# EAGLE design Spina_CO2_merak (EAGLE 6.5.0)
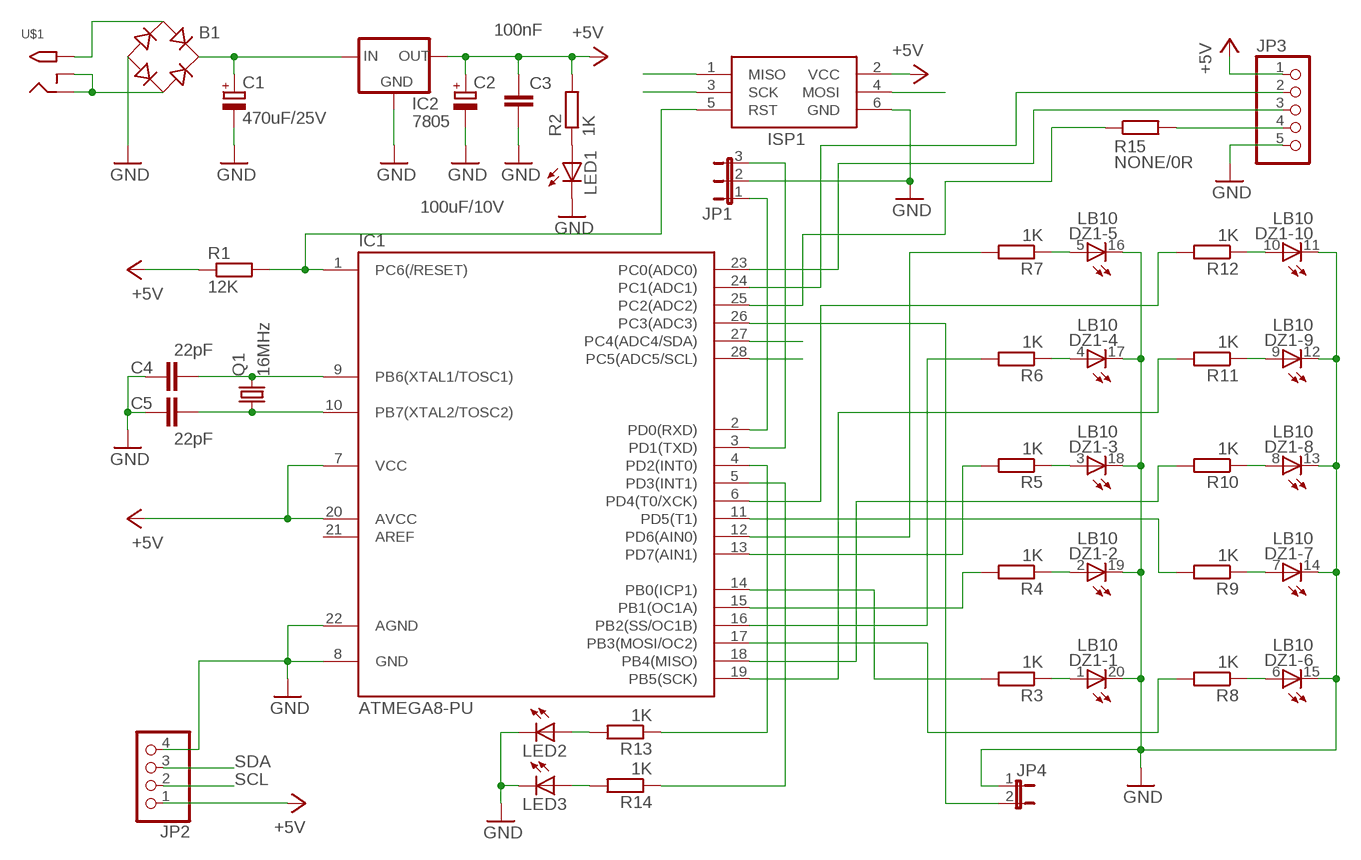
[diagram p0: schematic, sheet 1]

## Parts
B1  B-DIL  [B-DIL]
C1  470uF/25V  CPOL-EUE3.5-8  [E3,5-8]
C2  100uF/10V  CPOL-EUE2.5-6  [E2,5-6]
C3  100nF  C-EUC025_050-024X070  [C025_050-024X070]
C4  22pF  C-EUC025_050-024X070  [C025_050-024X070]
C5  22pF  C-EUC025_050-024X070  [C025_050-024X070]
DZ1  LB10  [LB10]
IC1  ATMEGA8-PU  [DIL28-3]
IC2  7805  78XXL  [78XXL]
ISP1  AVRISP-6  [AVRISP]
JP1  JP2E  [JP2]
JP2  PINHD-1X4  [1X04]
JP3  PINHD-1X5  [1X05]
JP4  JP1E  [JP1]
LED1  LED3MM  [LED3MM]
LED2  LED3MM  [LED3MM]
LED3  LED3MM  [LED3MM]
Q1  16MHz  CRYSTALHC49S  [HC49/S]
R1  12K  R-EU_0207/10  [0207/10]
R2  1K  R-EU_0207/10  [0207/10]
R3  1K  R-EU_0207/10  [0207/10]
R4  1K  R-EU_0207/10  [0207/10]
R5  1K  R-EU_0207/10  [0207/10]
R6  1K  R-EU_0207/10  [0207/10]
R7  1K  R-EU_0207/10  [0207/10]
R8  1K  R-EU_0207/10  [0207/10]
R9  1K  R-EU_0207/10  [0207/10]
R10  1K  R-EU_0207/10  [0207/10]
R11  1K  R-EU_0207/10  [0207/10]
R12  1K  R-EU_0207/10  [0207/10]
R13  1K  R-EU_0207/10  [0207/10]
R14  1K  R-EU_0207/10  [0207/10]
R15  NONE/0R  R-EU_R1206  [R1206]
U$1  2.1MMJACKTHM  [PJ-102A]

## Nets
+5V: C2.+ C3.1 IC1.7(VCC) IC1.20(AVCC) IC2.OUT ISP1.2(VCC) JP2.1 JP3.1 R1.1 R2.2
GND: B1.- C1.- C2.- C3.2 C4.1 C5.1 DZ1.11(-10:C) DZ1.12(-9:C) DZ1.13(-8:C) DZ1.14(-7:C) DZ1.15(-6:C) DZ1.16(-5:C) DZ1.17(-4:C) DZ1.18(-3:C) DZ1.19(-2:C) DZ1.20(-1:C) IC1.8(GND) IC1.22(AGND) IC2.GND ISP1.6(GND) JP1.2 JP2.4 JP3.5 JP4.1 LED1.K(C) LED2.K(C) LED3.K(C)
MISO: IC1.18(PB4(MISO)) ISP1.1(MISO) R10.2
MOSI: IC1.17(PB3(MOSI/OC2)) ISP1.4(MOSI) R8.2
N$1: B1.AC1 U$1.TIP
N$2: B1.AC2 U$1.RING U$1.RING_SW
N$3: B1.+ C1.+ IC2.IN
N$4: C4.2 IC1.9(PB6(XTAL1/TOSC1)) Q1.2
N$5: C5.2 IC1.10(PB7(XTAL2/TOSC2)) Q1.1
N$6: DZ1.5(-5:A) R7.1
N$7: IC1.1(PC6(/RESET)) ISP1.5(RST) R1.2
N$8: DZ1.10(-10:A) R12.1
N$9: LED1.A R2.1
N$10: IC1.2(PD0(RXD)) JP1.1
N$11: IC1.3(PD1(TXD)) JP1.3
N$12: DZ1.9(-9:A) R11.1
N$13: DZ1.8(-8:A) R10.1
N$14: DZ1.7(-7:A) R9.1
N$15: DZ1.2(-2:A) R4.1
N$16: DZ1.3(-3:A) R5.1
N$17: DZ1.4(-4:A) R6.1
N$18: DZ1.6(-6:A) R8.1
N$19: DZ1.1(-1:A) R3.1
N$20: IC1.24(PC1(ADC1)) JP3.2
N$21: IC1.23(PC0(ADC0)) JP3.3
N$22: IC1.25(PC2(ADC2)) R15.1
N$23: IC1.16(PB2(SS/OC1B)) R6.2
N$24: IC1.14(PB0(ICP1)) R3.2
N$25: IC1.15(PB1(OC1A)) R4.2
N$26: IC1.13(PD7(AIN1)) R5.2
N$27: IC1.11(PD5(T1)) R9.2
N$28: IC1.12(PD6(AIN0)) R7.2
N$29: IC1.6(PD4(T0/XCK)) R12.2
N$30: JP3.4 R15.2
N$31: IC1.26(PC3(ADC3)) JP4.2
N$33: LED2.A R13.2
N$34: LED3.A R14.2
N$35: IC1.4(PD2(INT0)) R13.1
N$36: IC1.5(PD3(INT1)) R14.1
SCK: IC1.19(PB5(SCK)) ISP1.3(SCK) R11.2
SCL: IC1.28(PC5(ADC5/SCL)) JP2.2
SDA: IC1.27(PC4(ADC4/SDA)) JP2.3
Unconnected: IC1.21(AREF)

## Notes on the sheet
- SDA
- SCL

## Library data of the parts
B1 = rectifier:B-DIL: RECTIFIER
C1 C2 = rcl:CPOL-EU: POLARIZED CAPACITOR, European symbol
C3-C5 = rcl:C-EU: CAPACITOR, European symbol
DZ1 = led:LB10: LED BLOCK 10-LED bar graph, DIL, Siemens
IC1 = atmega8:ATMEGA8-PU
IC2 = v-reg:78XXL: VOLTAGE REGULATOR
ISP1 = adafruit:AVRISP: AVR ISP HEADER Standard 6 pin header for AVR programming
JP1 = jumper:JP2E: JUMPER
JP2 = pinhead:PINHD-1X4: PIN HEADER
JP3 = pinhead:PINHD-1X5: PIN HEADER
JP4 = jumper:JP1E: JUMPER
LED1-LED3 = led:LED: LED
Q1 = crystal:CRYSTAL: CRYSTAL; OC_FARNELL: 1667008; OC_NEWARK: unknown
R1-R15 = rcl:R-EU_: RESISTOR, European symbol
U$1 = adafruit:2.1MMJACK: 2.1mm x 5.5mm THM DC jack with internal switch. Digikey part #PJ-102A, 4UCON part #05537 2.1mm x 5.5mm SMT DC jack with internal switch. Digikey part #PJ-002A-SMT, 4UCON part #03267 By microbuilder.eu & adafruit.com

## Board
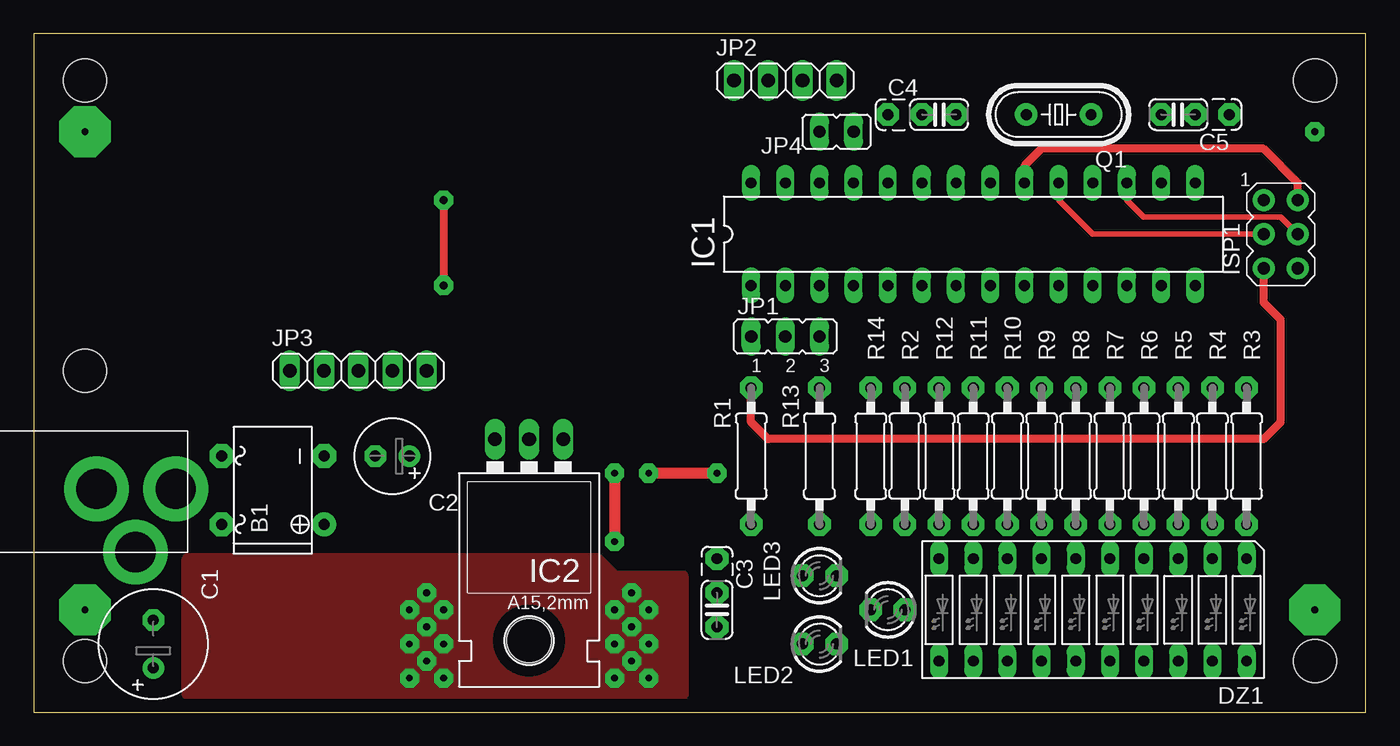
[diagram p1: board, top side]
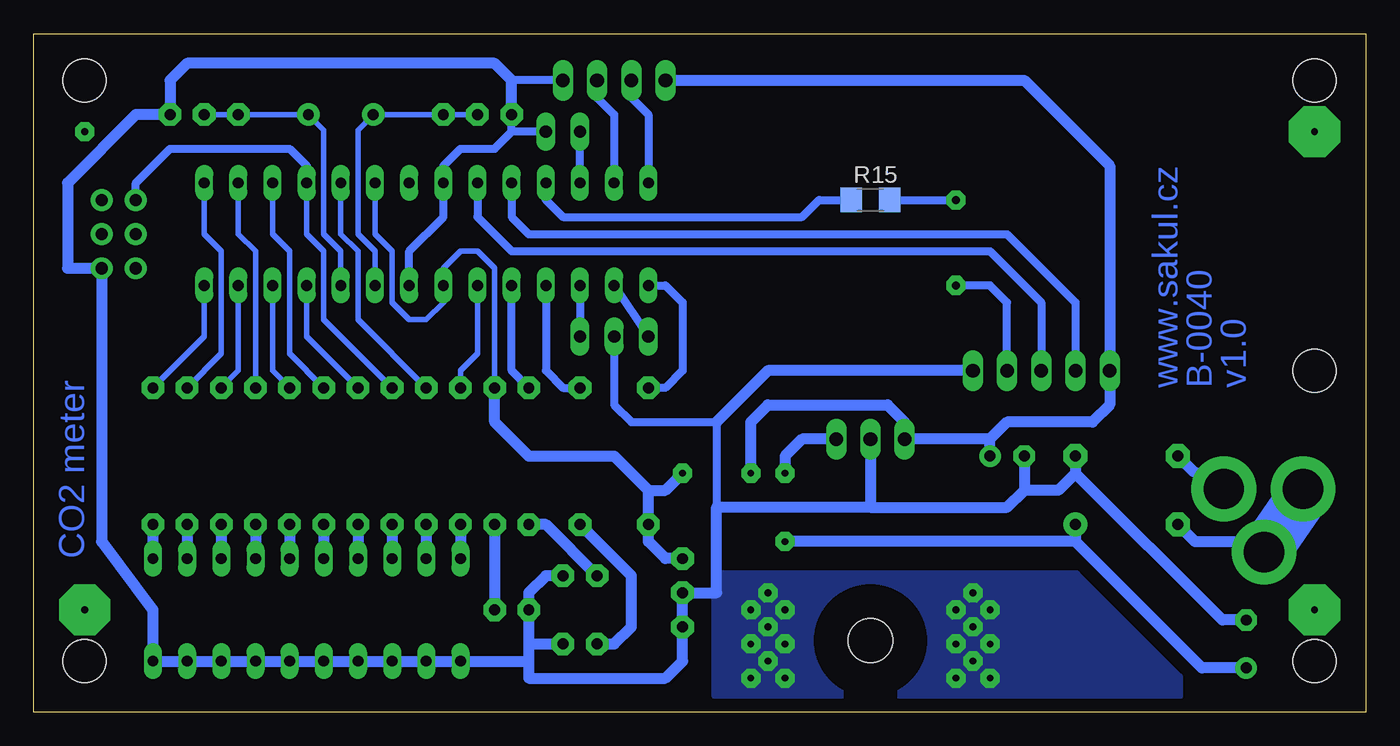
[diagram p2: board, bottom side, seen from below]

Size 99.04 x 50.47 mm. Coordinates in mm from the lower left corner, seen from the top.
Outline: 0,0 99.04,0 99.04,50.47 0,50.47 0,0
Copper layers (1*16): Top 0.035mm / dielectric 1.5mm / Bottom 0.035mm
Design rules "default": minimum track width 10mil, minimum drill 24mil, track to track 8mil, track to pad 8mil, pad to pad 8mil, via to via 8mil, smd to smd 8mil, copper to edge 40mil, drill to drill 8mil, minimum pad ring 10mil, minimum via ring 8mil, stop-mask expansion 4mil, vias tented up to drill 0mil, thermal gap 10mil
Holes 3.2 mm at 3.81,3.81 95.25,3.81 95.25,46.99 3.81,46.99 3.81,25.4

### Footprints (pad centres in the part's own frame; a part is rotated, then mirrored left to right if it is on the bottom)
B-DIL = drill 0.813 pad 1.778: + -2.54,-3.81 | drill 0.813 pad 1.778 octagon: - 2.54,-3.81; AC1 2.54,3.81; AC2 -2.54,3.81
E3,5-8 = drill 0.813 pad 1.6: + -1.778,0 | drill 0.813 pad 1.6 octagon: - 1.778,0
E2,5-6 = drill 0.813 pad 1.6: + -1.27,0 | drill 0.813 pad 1.6 octagon: - 1.27,0
C025_050-024X070 = drill 0.813 pad 1.676 octagon: 1 -3.81,0; 2 -1.27,0; 3 1.27,0
LB10 = drill 0.813 long: 1 -11.43,-3.81; 2 -8.89,-3.81; 3 -6.35,-3.81; 4 -3.81,-3.81; 5 -1.27,-3.81; 6 1.27,-3.81; 7 3.81,-3.81; 8 6.35,-3.81; 9 8.89,-3.81; 10 11.43,-3.81; 11 11.43,3.81; 12 8.89,3.81; 13 6.35,3.81; 14 3.81,3.81; 15 1.27,3.81; 16 -1.27,3.81; 17 -3.81,3.81; 18 -6.35,3.81; 19 -8.89,3.81; 20 -11.43,3.81
DIL28-3 = drill 0.813 long: 1 -16.51,-3.81; 2 -13.97,-3.81; 3 -11.43,-3.81; 4 -8.89,-3.81; 5 -6.35,-3.81; 6 -3.81,-3.81; 7 -1.27,-3.81; 8 1.27,-3.81; 9 3.81,-3.81; 10 6.35,-3.81; 11 8.89,-3.81; 12 11.43,-3.81; 13 13.97,-3.81; 14 16.51,-3.81; 15 16.51,3.81; 16 13.97,3.81; 17 11.43,3.81; 18 8.89,3.81; 19 6.35,3.81; 20 3.81,3.81; 21 1.27,3.81; 22 -1.27,3.81; 23 -3.81,3.81; 24 -6.35,3.81; 25 -8.89,3.81; 26 -11.43,3.81; 27 -13.97,3.81; 28 -16.51,3.81
78XXL = drill 1.016 long: GND 0,-3.81; IN -2.54,-3.81; OUT 2.54,-3.81 | hole 3.302: 0,11.176
AVRISP = drill 0.9 pad 1.626: 1 -1.27,2.54; 2 1.27,2.54; 3 -1.27,0; 4 1.27,0; 5 -1.27,-2.54; 6 1.27,-2.54
JP2 = drill 0.914 long: 1 -2.54,0; 2 0,0; 3 2.54,0
1X04 = drill 1.016 long: 1 -3.81,0; 2 -1.27,0; 3 1.27,0; 4 3.81,0
1X05 = drill 1.016 long: 1 -5.08,0; 2 -2.54,0; 3 0,0; 4 2.54,0; 5 5.08,0
JP1 = drill 0.914 long: 1 0,-1.27; 2 0,1.27
LED3MM = drill 0.813 pad 1.676 octagon: A -1.27,0; K 1.27,0
HC49/S = drill 0.813 pad 1.676: 1 -2.413,0; 2 2.413,0
0207/10 = drill 0.813 pad 1.676 octagon: 1 -5.08,0; 2 5.08,0
R1206 = smd 1.6 x 1.803: 1 -1.422,0; 2 1.422,0
PJ-102A = drill 3 pad 4.8: RING 0.1,-3.39; RING_SW -4.6,-6.29; TIP 0.1,-9.29

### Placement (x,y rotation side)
B1  17.78,16.51 90 top
C1  8.89,5.08 90 top
C2  26.67,19.05 180 top
C3  50.8,7.62 270 top
C4  67.31,44.45 0 top
C5  85.09,44.45 180 top
DZ1  78.74,7.62 180 top
IC1  69.85,35.56 0 top
IC2  36.83,16.51 180 top
ISP1  92.71,35.56 0 top
JP1  55.88,27.94 0 top
JP2  55.88,46.99 0 top
JP3  24.13,25.4 0 top
JP4  59.69,43.18 90 top
LED1  63.5,7.62 180 top
LED2  58.42,5.08 0 top
LED3  58.42,10.16 0 top
Q1  76.2,44.45 180 top
R1  53.34,19.05 90 top
R2  64.77,19.05 90 top
R3  90.17,19.05 90 top
R4  87.63,19.05 90 top
R5  85.09,19.05 90 top
R6  82.55,19.05 90 top
R7  80.01,19.05 90 top
R8  77.47,19.05 90 top
R9  74.93,19.05 90 top
R10  72.39,19.05 90 top
R11  69.85,19.05 90 top
R12  67.31,19.05 90 top
R13  58.42,19.05 270 top
R14  62.23,19.05 270 top
R15  36.83,38.1 0 bottom
U$1  1.27,16.51 90 top

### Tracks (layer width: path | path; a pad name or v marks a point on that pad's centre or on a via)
+5V  (via drill 0.5 pad 1.42)
  Top 0.61: ISP1.2 93.98,39.37 91.44,41.91 74.93,41.91 73.66,40.64 IC1.20
  Top 0.813: v50.8,17.78 v45.72,17.78
  Bottom 0.406: IC1.20 73.66,35.56 72.39,34.29 72.39,30.48 71.12,29.21 69.85,29.21 68.58,30.48 IC1.7 68.58,33.02 67.31,34.29 66.04,34.29 64.77,33.02 64.77,21.59
  Bottom 0.813: R2.2 64.77,21.59 62.23,19.05 55.88,19.05 53.34,16.51 | JP2.1 25.4,46.99 19.05,40.64 JP3.1 19.05,22.86 20.32,21.59 26.67,21.59 27.94,20.32 | C2.+ 27.94,20.32 | 27.94,20.32 IC2.OUT 34.29,21.59 35.56,22.86 44.45,22.86 45.72,21.59 v45.72,17.78 | C3.1 52.07,11.43 53.34,12.7 R1.1 53.34,16.51 | 53.34,16.51 52.07,16.51 v50.8,17.78
GND  (via drill 0.5 pad 1.42)
  Bottom 0.61: 63.5,43.18 64.77,41.91 67.31,41.91 68.58,40.64 IC1.22 68.58,36.83 71.12,34.29 IC1.8 | 63.5,43.18 C4.1 | JP4.1 63.5,43.18 | JP2.4 63.5,46.99 | JP1.2 55.88,22.86 54.61,21.59 48.26,21.59 48.26,15.24
  Bottom 0.813: 62.23,3.81 DZ1.11 DZ1.12 DZ1.13 DZ1.14 DZ1.15 DZ1.16 DZ1.17 DZ1.18 DZ1.19 DZ1.20 90.17,7.62 93.98,12.7 ISP1.6 96.52,33.02 96.52,39.37 91.44,44.45 C5.1 88.9,46.99 87.63,48.26 64.77,48.26 63.5,46.99 C4.1 | 62.23,5.08 LED2.K | 62.23,5.08 LED1.K 62.23,8.89 60.96,10.16 LED3.K | 62.23,5.08 62.23,3.81 | 62.23,3.81 62.23,2.54 52.07,2.54 50.8,3.81 C3.2 48.26,8.89 48.26,15.24 36.83,15.24 | C1.- 10.67,6.86 21.59,17.78 | B1.- 21.59,17.78 | 21.59,17.78 22.86,16.51 25.4,16.51 | IC2.GND 36.83,15.24 | 36.83,15.24 26.67,15.24 25.4,16.51 | C2.- 25.4,16.51 | JP3.5 44.45,25.4 48.26,21.59
  other vias: 29.21,8.89 27.94,7.62 30.48,7.62 29.21,6.35 27.94,5.08 30.48,5.08 29.21,3.81 30.48,2.54 27.94,2.54 44.45,8.89 43.18,7.62 45.72,7.62 44.45,6.35 45.72,5.08 43.18,5.08 44.45,3.81 45.72,2.54 43.18,2.54
  pour Bottom: 13.97,1.27 13.97,2.54 21.59,10.16 48.26,10.16 48.26,1.27
  pour Top: 11.43,11.43 41.91,11.43 43.18,10.16 48.26,10.16 48.26,1.27 11.43,1.27
MISO
  Bottom 0.406: IC1.18 78.74,35.56 77.47,34.29 77.47,29.21 R10.2
  Bottom 0.61: ISP1.1 91.44,39.37 88.9,41.91 80.01,41.91 78.74,40.64 IC1.18
MOSI
  Top 0.406: ISP1.4 92.71,36.83 82.55,36.83 81.28,38.1 IC1.17
  Bottom 0.406: IC1.17 81.28,35.56 80.01,34.29 80.01,26.67 R8.2
N$1
  Bottom 0.813: U$1.TIP 12.8,17.88 B1.AC1
N$2
  Bottom 0.813: B1.AC2 12.7,12.7 8.04,12.7 U$1.RING_SW
  Bottom 3.81: U$1.RING 4.66,16.08 U$1.RING_SW
N$3  (via drill 0.5 pad 1.42)
  Top 0.813: v43.18,17.78 v43.18,12.7
  Bottom 0.813: C1.+ 12.19,3.3 21.59,12.7 | IC2.IN 41.91,20.32 43.18,19.05 v43.18,17.78 | B1.+ 21.59,12.7 | 21.59,12.7 v43.18,12.7
N$4
  Bottom 0.406: C4.2 Q1.2 74.93,43.31 74.93,35.56 73.66,34.29 IC1.9
N$5
  Bottom 0.406: IC1.10 76.2,34.29 77.47,35.56 77.47,43.31 Q1.1 C5.2
N$6
  Bottom 0.813: R7.1 DZ1.5
N$7
  Top 0.61: R1.2 53.34,21.59 54.61,20.32 91.44,20.32 92.71,21.59 92.71,29.21 91.44,30.48 ISP1.5
  Bottom 0.61: IC1.1 52.07,31.75 50.8,30.48 50.8,25.4 52.07,24.13 R1.2
N$8
  Bottom 0.813: R12.1 DZ1.10
N$9
  Bottom 0.813: R2.1 LED1.A
N$10
  Bottom 0.61: IC1.2 JP1.1
N$11
  Bottom 0.61: IC1.3 JP1.3
N$12
  Bottom 0.813: R11.1 DZ1.9
N$13
  Bottom 0.813: R10.1 DZ1.8
N$14
  Bottom 0.813: R9.1 DZ1.7
N$15
  Bottom 0.813: R4.1 DZ1.2
N$16
  Bottom 0.813: R5.1 DZ1.3
N$17
  Bottom 0.813: R6.1 DZ1.4
N$18
  Bottom 0.813: R8.1 DZ1.6
N$19
  Bottom 0.813: R3.1 DZ1.1
N$20
  Bottom 0.61: IC1.24 63.5,36.83 62.23,35.56 26.67,35.56 21.59,30.48 JP3.2
N$21
  Bottom 0.61: IC1.23 66.04,36.83 63.5,34.29 27.94,34.29 24.13,30.48 JP3.3
N$22
  Bottom 0.61: IC1.25 60.96,38.1 59.69,36.83 41.91,36.83 40.64,38.1 R15.1
N$23
  Bottom 0.406: IC1.16 83.82,35.56 82.55,34.29 R6.2
N$24
  Bottom 0.406: IC1.14 86.36,27.94 R3.2
N$25
  Bottom 0.406: IC1.15 86.36,35.56 85.09,34.29 85.09,26.67 R4.2
N$26
  Bottom 0.406: IC1.13 83.82,25.4 R5.2
N$27
  Bottom 0.406: IC1.11 78.74,27.94 R9.2
N$28
  Bottom 0.406: IC1.12 81.28,25.4 R7.2
N$29
  Bottom 0.406: IC1.6 66.04,26.67 67.31,25.4 R12.2
N$30  (via drill 0.6 pad 1.42)
  Top 0.61: v30.48,38.1 v30.48,31.75
  Bottom 0.61: R15.2 v30.48,38.1 | JP3.4 26.67,30.48 27.94,31.75 v30.48,31.75
N$31
  Bottom 0.61: IC1.26 JP4.2
N$32  (via drill 0.5 pad 3.81)
  other vias: 3.81,7.62
N$33
  Bottom 0.813: LED2.A 55.88,5.08 54.61,6.35 54.61,10.16 R13.2
N$34
  Bottom 0.813: LED3.A 60.96,13.97 R14.2
N$35
  Bottom 0.61: IC1.4 60.96,25.4 59.69,24.13 R13.1
N$36
  Bottom 0.61: R14.1 63.5,25.4 IC1.5
N$37  (via drill 0.5 pad 3.81)
  other vias: 95.25,7.62
N$38  (via drill 0.5 pad 3.81)
  other vias: 3.81,43.18
N$39  (via drill 0.5 pad 1.42)
  other vias: 95.25,43.18
SCK
  Top 0.406: ISP1.3 78.74,35.56 76.2,38.1 IC1.19
  Bottom 0.406: IC1.19 76.2,35.56 74.93,34.29 74.93,29.21 R11.2
SCL
  Bottom 0.61: JP2.2 54.61,45.72 53.34,44.45 IC1.28
SDA
  Bottom 0.61: JP2.3 57.15,45.72 55.88,44.45 IC1.27

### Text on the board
Bottom: v1.0 | B-0040 | www.sakul.cz | CO2 meter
